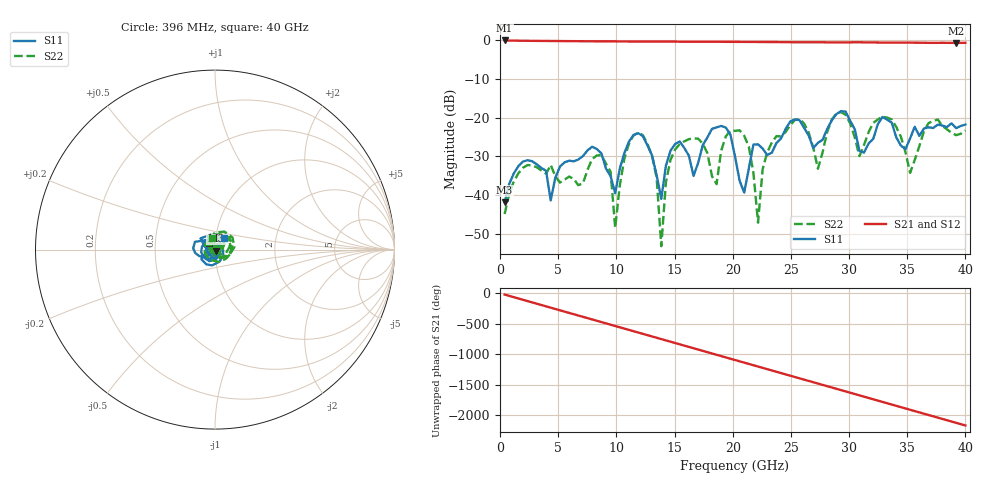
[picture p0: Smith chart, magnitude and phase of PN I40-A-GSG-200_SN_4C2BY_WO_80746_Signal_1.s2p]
!  2-Port S-parameters as saved by WinCal
!VAR DATE=05-13-2004  08:01:21
!VAR OPNAME=bhollow
# Hz S RI R 50.00
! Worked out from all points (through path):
!   101 points, 396 MHz to 40 GHz, reference 50 ohm
!   highest |S21| = -0.06 dB at 396 MHz (marker M1); lowest = -0.7 dB at 39.21 GHz (marker M2)
!   group delay of S21, straight-line fit = 151 ps
!   lowest |S11| = -41.8 dB at 396 MHz (marker M3), VSWR 1.02, Z = 50.5 - j0.67 ohm
!   |S11| at or under -10 dB: start of sweep to end of sweep
!   |S22| runs from -53.1 to -18.5 dB; largest |S21 - S12| = 0
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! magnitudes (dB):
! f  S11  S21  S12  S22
! 396 MHz  -41.8  -0.1  -0.1  -44.9
! 2.376 GHz  -31.0  -0.1  -0.1  -32.2
! 4.356 GHz  -41.3  -0.2  -0.2  -32.2
! 7.129 GHz  -29.9  -0.3  -0.3  -36.9
! 8.713 GHz  -29.2  -0.3  -0.3  -29.6
! 9.901 GHz  -39.5  -0.3  -0.3  -48.4
! 10.69 GHz  -29.1  -0.3  -0.3  -30.5
! 12.28 GHz  -24.8  -0.3  -0.3  -24.5
! 13.47 GHz  -34.9  -0.3  -0.3  -35.5
! 13.86 GHz  -40.9  -0.3  -0.3  -53.1
! 15.05 GHz  -26.8  -0.4  -0.4  -28.2
! 16.63 GHz  -35.0  -0.4  -0.4  -25.3
! 18.61 GHz  -22.5  -0.4  -0.4  -37.1
! 20.2 GHz  -30.0  -0.4  -0.4  -23.4
! 20.99 GHz  -39.3  -0.4  -0.4  -24.7
! 22.18 GHz  -26.9  -0.5  -0.5  -47.1
! 23.76 GHz  -26.5  -0.5  -0.5  -24.7
! 26.93 GHz  -27.8  -0.5  -0.5  -27.8
! 33.66 GHz  -21.2  -0.6  -0.6  -20.4
! 35.25 GHz  -25.3  -0.6  -0.6  -34.2
! 39.21 GHz  -22.7  -0.7  -0.7  -24.5
! 40 GHz  -21.8  -0.7  -0.7  -23.3
